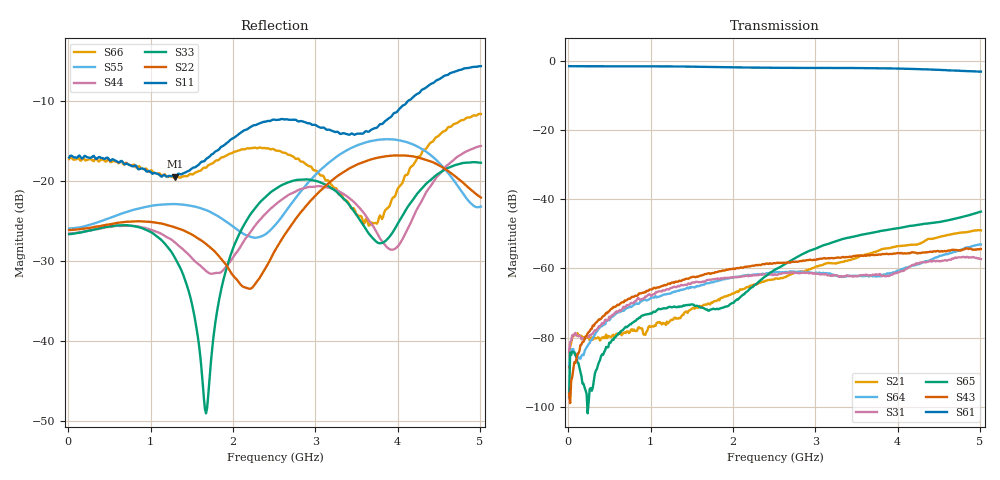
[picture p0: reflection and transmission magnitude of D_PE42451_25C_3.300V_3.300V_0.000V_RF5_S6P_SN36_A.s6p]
! Device ID: PE42451
! Serial: 36
! Insertion: A
! Temp: 25C
! VDD: 3.300
! Control_Hi: 100.000
! Control_Lo: 0.000
! Logic State: RF5
! Port 1: RFC
! Port 2: RF1
! Port 3: RF2
! Port 4: RF3
! Port 5: RF4
! Port 6: RF5
! V1 = 3.30
! V2 = 0.00
! V3 = 3.30
! V4 = 0.00
! IDD: 1.634180e-05
#  Hz  S  RI  R  50
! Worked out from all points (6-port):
!   401 points, 10 MHz to 5.01 GHz, reference 50 ohm
!   strongest paths, dB at 10 MHz, 1.26 GHz, 2.51 GHz, 3.76 GHz, 5.01 GHz:
!     S61: -1.5, -1.5, -1.9, -2.1, -3.0
!     S43: -96.2, -64.1, -58.5, -56.1, -54.4
!     S65: -97.3, -71.2, -60.3, -49.3, -43.5
!     S31: -84.3, -65.6, -61.7, -61.9, -57.3
!     S64: -87.9, -66.9, -61.1, -62.2, -53.1
!     S21: -88.7, -74.9, -62.9, -54.9, -49.0
!   lowest |S11| = -19.5 dB at 1.298 GHz (marker M1), VSWR 1.24, Z = 54.3 - j10.2 ohm
!   |S11| at or under -10 dB: start of sweep to 4.132 GHz
